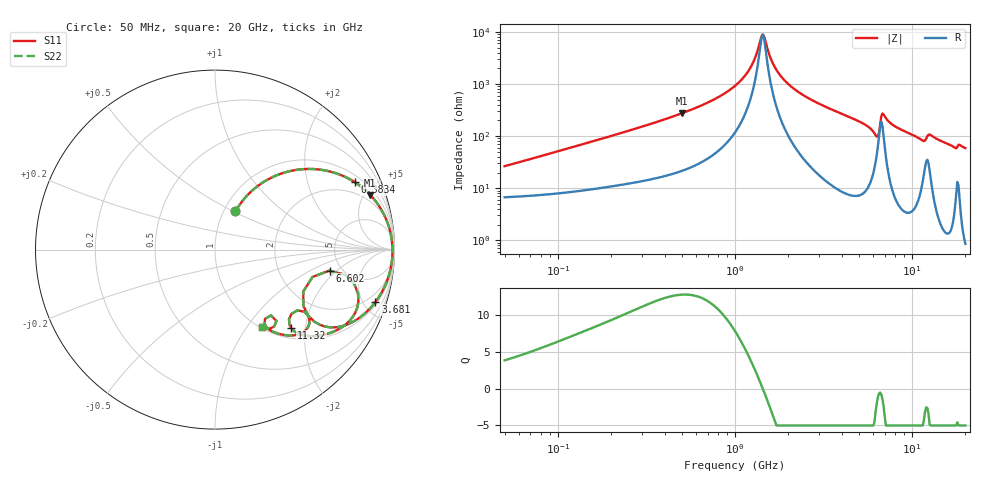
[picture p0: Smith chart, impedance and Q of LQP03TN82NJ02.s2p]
!Murata Part Number: LQP03TN82NJ02
!These Parameters are Measured in Series Mode Connection
!  o--[Z]--o
!Port1  Port2
!  o-------o
!Freq. Start=50[MHz] Stop=20[GHz], 401[Steps]
# Hz S RI R 50
!Freq.(Hz) S11(Real) S11(Imag) S21(Real) S21(Imag) S12(Real) S12(Imag) S22(Real) S22(Imag)
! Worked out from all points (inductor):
!   401 points, 50 MHz to 20 GHz, reference 50 ohm
!   read as one part in series: L = 80.8 nH near 51.52 MHz
!   highest Q = 12.7 at 502.1 MHz (marker M1), where L = 86.8 nH
!   self-resonance near 1.433 GHz
!   S11 on the Smith chart (normalised r, x): 50 MHz: 1.13, +0.51; 383.4 MHz: 1.33, +3.98; 3.681 GHz: 1.20, -6.05; 6.602 GHz: 4.00, -1.61; 11.32 GHz: 1.21, -1.67; 20 GHz: 1.02, -1.18
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5e7  0.1137 0.2125  0.8863 -0.2125  0.8863 -0.2125  0.1137 0.2125
1.364002e8  0.3421 0.4135  0.6579 -0.4135  0.6579 -0.4135  0.3421 0.4135
3.721004e8  0.7698 0.3814  0.2302 -0.3814  0.2302 -0.3814  0.7698 0.3814
3.834161e8  0.7806 0.3746  0.2194 -0.3746  0.2194 -0.3746  0.7806 0.3746
5.020686e8  0.8646 0.3051  0.1354 -0.3051  0.1354 -0.3051  0.8646 0.3051
1e9  0.9754 0.1036  0.0246 -0.1036  0.0246 -0.1036  0.9754 0.1036
1.214974e9  0.9857 0.0475  0.0143 -0.0475  0.0143 -0.0475  0.9857 0.0475
1.432596e9  0.9889 0.000354  0.0111 -0.000354  0.0111 -0.000354  0.9889 0.000354
1.639343e9  0.988 -0.0385  0.012 0.0385  0.012 0.0385  0.988 -0.0385
1.820564e9  0.9849 -0.069  0.0151 0.069  0.0151 0.069  0.9849 -0.069
2.728004e9  0.9511 -0.1927  0.0489 0.1927  0.0489 0.1927  0.9511 -0.1927
3.680849e9  0.8938 -0.2918  0.1062 0.2918  0.1062 0.2918  0.8938 -0.2918
5.856089e9  0.6382 -0.4327  0.3618 0.4327  0.3618 0.4327  0.6382 -0.4327
6.311513e9  0.4922 -0.3126  0.5078 0.3126  0.5078 0.3126  0.4922 -0.3126
6.601595e9  0.638 -0.1166  0.362 0.1166  0.362 0.1166  0.638 -0.1166
6.905011e9  0.7971 -0.2466  0.2029 0.2466  0.2029 0.2466  0.7971 -0.2466
7.442007e9  0.7562 -0.3894  0.2438 0.3894  0.2438 0.3894  0.7562 -0.3894
9.316812e9  0.5838 -0.4789  0.4162 0.4789  0.4162 0.4789  0.5838 -0.4789
1.131968e10  0.424 -0.4362  0.576 0.4362  0.576 0.4362  0.424 -0.4362
1.201863e10  0.4583 -0.3391  0.5417 0.3391  0.5417 0.3391  0.4583 -0.3391
1.276073e10  0.5177 -0.4337  0.4823 0.4337  0.4823 0.4337  0.5177 -0.4337
2e10  0.2603 -0.4316  0.7397 0.4316  0.7397 0.4316  0.2603 -0.4316
